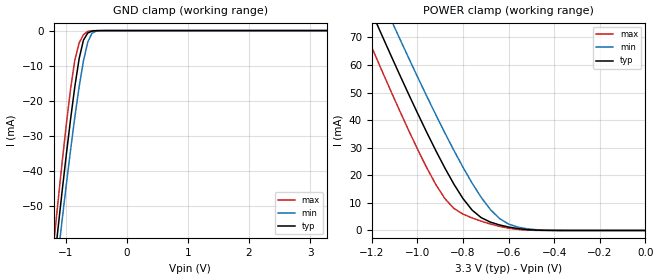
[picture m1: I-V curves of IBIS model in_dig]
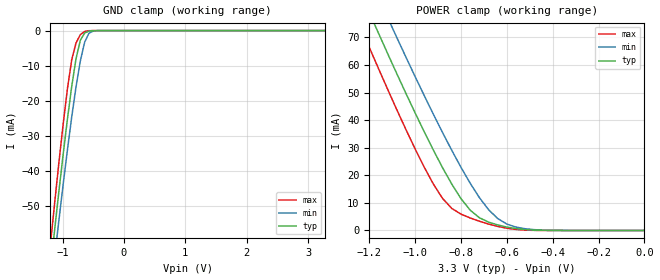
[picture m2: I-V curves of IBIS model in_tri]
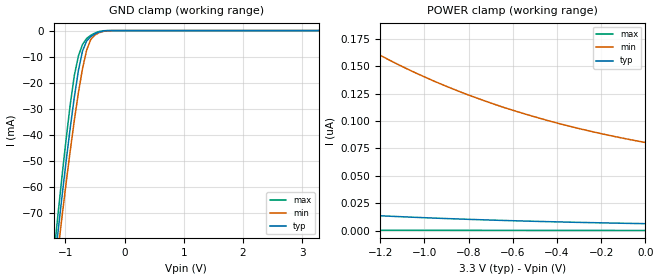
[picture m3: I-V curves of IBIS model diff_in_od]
| Integrated Devices Technolgy, Inc
[Ibis Ver]   4.1
[File Name]   9zxl0853e.ibs
[File Rev]   1.0
[Date]   Thrusday October 22, 2020
[Source]   Integrated Devices Technolgy, Inc.
[Notes]   Rev 1.0 created by LFP
|   Derived from 9zxl0832e
[Disclaimer] Integrated Device Technology, Inc. ("IDT") hereby grants the
   user of this IBIS model a non-exclusive, nontransferable
   license to use this IBIS model under the following terms. The
   user is granted this license only to use the IBIS model and is
   not granted rights to sell, copy (except as needed to run the
   IBIS model), rent, lease or sub-license the IBIS model in
   whole or in part, or in modified form to anyone. The User may
   modify the IBIS model to suit its specific applications, but
   rights to derivative works and such modifications shall belong
   to IDT. This IBIS model is provided on an AS IS" basis and IDT
   makes absolutely no warranty with respect to the information
   contained herein. IDT DISCLAIMS AND CUSTOMER WAIVES ALL
   WARRANTIES, EXPRESS AND IMPLIED, INCLUDING WARRANTIES OF
   MERCHANTABILITY AND FITNESS FOR A PARTICULAR PURPOSE. THE
   ENTIRE RISK AS TO QUALITY AND PERFORMANCE IS WITH THE USER
   ACCORDINGLY, IN NO EVENT SHALL IDT BE LIABLE FOR ANY DIRECT OR
   INDIRECT DAMAGES, WHETHER IN CONTRACT OR TORT, INCLUDING ANY
   LOST PROFITS OR OTHER INCIDENTAL, CONSEQUENTIAL, EXEMPLARY, OR
   PUNITIVE DAMAGES ARISING OUT OF THE USE OR APPLICATION OF THE
   IBIS model. Further, IDT reserves the right to make changes
   without notice to any product herein to improve reliability,
   function, or design. IDT does not convey any license under
   patent rights or any other intellectual property rights,
   including those of third parties. IDT is not obligated to
   provide maintenance or support for the licensed IBIS model.
   (C) Copyright Integrated Device Technology, Inc. 2016 All
   rights reserved
|   COMPONENT: 9zxl0853e
[Component]   9zxl0853e
[Manufacturer]   Integrated Device Technology, Inc.
[Package]
| variable   typ   min   max
R_pkg   81.10m   62.20m   100.00m
L_pkg   6.70nH   4.90nH   8.50nH
C_pkg   0.53pF   0.21pF   0.85pF
[Pin]   signal_name   model_name   R_pin   L_pin   C_pin
1   CKPWRGD_PD#   in_dig
2   VDDR   POWER
3   DIF_IN   diff_in_od
4   DIF_IN#   diff_in_od
5   vSADR0_tri   in_dig
6   SMBDAT   sda_od
7   SMBCLK   scl_od
8   vSADR1_tri   in_dig
9   FBOUT_NC#   NC
10   FBOUT_NC   NC
11   VDD   POWER
12   OE_0#   in_dig
13   DIF_0   diff_out
14   DIF_0#   diff_out
15   VDD   POWER
16   DIF_1   diff_out
17   DIF_1#   diff_out
18   OE_1#   in_dig
19   VDD   POWER
20   NC   NC
21   DIF_2   diff_out
22   DIF_2#   diff_out
23   OE_2#   in_dig
24   OE_3#   in_dig
25   DIF_3   diff_out
26   DIF_3#   diff_out
27   VDD   POWER
28   DIF_4   diff_out
29   DIF_4#   diff_out
30   OE_4#   in_dig
31   OE_5#   in_dig
32   DIF_5   diff_out
33   DIF_5#   diff_out
34   VDD   POWER
35   DIF_6   diff_out
36   DIF_6#   diff_out
37   OE_6#   in_dig
38   VDD   POWER
39   DIF_7   diff_out
40   DIF_7#   diff_out
41   OE_7#   in_dig
42   VDD   POWER
43   NC   NC
44   VDDA   POWER
45   NC   NC
46   SMB_WRTLOCK   in_dig
47   100M_133M#   in_dig
48   HBW_BYP_LOBW#  in_tri
49   EPAD   GND
[Diff Pin]   inv_pin   vdiff   tdelay_typ
3   4   NA   NA
13   14   NA   NA
16   17   NA   NA
21   22   NA   NA
25   26   NA   NA
28   29   NA   NA
32   33   NA   NA
35   36   NA   NA
39   40   NA   NA
| Models and submodels in the file (6): in_dig (Input), in_tri (Input), diff_in_od (Input), sda_od (I/O_open_drain), scl_od (Input), diff_out (Output)
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|   Model in_dig
[Model]  in_dig
Model_type Input
Polarity   Non-Inverting
Vinl =   0.8000V
Vinh =   2.0000V
C_comp   2.1000pF   2.1000pF   2.1000pF
[Temperature Range]   25.0000   85.0000   -40.0000
[Voltage Range]   3.3000V   3.1350V   3.4650V
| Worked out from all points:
|   GND clamp passes 1 mA (typ) near -0.65 V on its own axis
|   POWER clamp passes 1 mA (typ) near -0.58 V on its own axis
[GND_clamp]
|Voltage   I(typ)   I(min)   I(max)
-3.3V     -444.4mA   -436.3mA   -455.2mA
-1.2V     -68.37mA   -75.7mA    -61.37mA
-1.13V    -56.99mA   -64.8mA    -49.35mA
-1.06V    -45.92mA   -54.16mA   -37.72mA
-920mV    -25.14mA   -33.91mA   -16.51mA
-850mV    -15.84mA   -24.53mA   -8.255mA
-780mV    -7.95mA    -15.96mA   -3.499mA
-710mV    -2.728mA   -8.626mA   -1.156mA
-640mV    -697.7uA   -3.286mA   -240.6uA
-570mV    -146.6uA   -751uA     -34.01uA
-430mV    -3.844uA   -23.08uA   -279.3nA
3.28V     213.4pA    44.16nA    205.9pA
[POWER_clamp]
|Voltage   I(typ)   I(min)   I(max)
-3.28V    509.3mA    515.8mA    504.9mA
-1.24V    86.61mA    99.33mA    74.1mA
-1.16V    71.55mA    84.5mA     58.72mA
-1.12V    64.14mA    77.19mA    51.18mA
-1.08V    56.84mA    69.96mA    43.78mA
-960mV    35.71mA    48.84mA    22.88mA
-880mV    22.69mA    35.43mA    11.57mA
-840mV    16.77mA    29.02mA    7.979mA
-760mV    7.367mA    17.14mA    4.53mA
-640mV    2.005mA    4.321mA    1.477mA
-480mV    131.2uA    293.3uA    37.64uA
0V        220.8pA    394.5pA    228.5pA
|   Model in_tri
[Model]  in_tri
Model_type Input
Polarity   Non-Inverting
Vinl =   0.8000V
Vinh =   2.0000V
C_comp   2.1400pF   2.1400pF   2.1400pF
[Temperature Range]   25.0000   85.0000   -40.0000
[Voltage Range]   3.3000V   3.1350V   3.4650V
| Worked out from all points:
|   GND clamp passes 1 mA (typ) near -0.65 V on its own axis
|   POWER clamp passes 1 mA (typ) near -0.58 V on its own axis
[GND_clamp]
|Voltage   I(typ)   I(min)   I(max)
-3.3V     -444.4mA   -436.3mA   -455.2mA
-1.2V     -68.37mA   -75.7mA    -61.37mA
-1.13V    -56.99mA   -64.8mA    -49.35mA
-1.06V    -45.92mA   -54.16mA   -37.72mA
-920mV    -25.14mA   -33.91mA   -16.51mA
-850mV    -15.84mA   -24.53mA   -8.255mA
-780mV    -7.95mA    -15.96mA   -3.499mA
-710mV    -2.728mA   -8.625mA   -1.156mA
-640mV    -697.7uA   -3.286mA   -240.6uA
-570mV    -146.6uA   -751uA     -34.01uA
-430mV    -3.844uA   -23.08uA   -279.3nA
3.28V     213.4pA    44.16nA    205.9pA
[POWER_clamp]
|Voltage   I(typ)   I(min)   I(max)
-3.28V    509.3mA    515.8mA    504.9mA
-1.24V    86.61mA    99.33mA    74.1mA
-1.16V    71.55mA    84.5mA     58.72mA
-1.12V    64.14mA    77.19mA    51.18mA
-1.08V    56.84mA    69.96mA    43.78mA
-960mV    35.71mA    48.84mA    22.88mA
-880mV    22.69mA    35.43mA    11.57mA
-840mV    16.77mA    29.02mA    7.979mA
-760mV    7.367mA    17.14mA    4.53mA
-640mV    2.005mA    4.321mA    1.477mA
-480mV    131.2uA    293.3uA    37.64uA
0V        220.8pA    394.5pA    228.4pA
|   Model diff_in_od
[Model]  diff_in_od
Model_type Input
Polarity   Non-Inverting
Vinl =   0.3000V
Vinh =   0.5000V
C_comp   3.5000pF   3.5000pF   3.5000pF
[Temperature Range]   25.0000   85.0000   -40.0000
[Voltage Range]   3.3000V   3.1350V   3.4650V
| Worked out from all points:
|   GND clamp passes 1 mA (typ) near -0.47 V on its own axis
[GND_clamp]
|Voltage   I(typ)   I(min)   I(max)
-3.3V     -581.4mA   -566.8mA   -600.3mA
-1.2V     -92.9mA    -99.3mA    -87.17mA
-1.13V    -78.34mA   -85.45mA   -71.6mA
-1.06V    -64.19mA   -71.96mA   -56.52mA
-920mV    -37.64mA   -46.39mA   -28.76mA
-850mV    -25.69mA   -34.6mA    -17.37mA
-780mV    -15.32mA   -23.82mA   -9.726mA
-710mV    -7.779mA   -14.52mA   -5.31mA
-640mV    -3.984mA   -7.427mA   -3.004mA
-500mV    -1.282mA   -1.675mA   -939.5uA
-220mV    -3.662uA   -14.35uA   -357.2nA
3.28V     6.54nA     86.14nA    391.5pA
[POWER_clamp]
|Voltage   I(typ)   I(min)   I(max)
-3.28V    57.48nA    654.6nA    1.522nA
-2.84V    43.19nA    492.3nA    1.256nA
-2.4V     32.05nA    365.8nA    1.04nA
-1.92V    22.9nA     262.2nA    852pA
-1.4V     15.85nA    182.8nA    693.7pA
-1.12V    13.05nA    151.5nA    623.8pA
-960mV    11.71nA    136.6nA    587.9pA
-800mV    10.54nA    123.6nA    554.6pA
-640mV    9.52nA     112.3nA    523.5pA
-440mV    8.427nA    100.3nA    487.7pA
-240mV    7.511nA    90.3nA     454.6pA
0V        6.607nA    80.43nA    417.9pA
